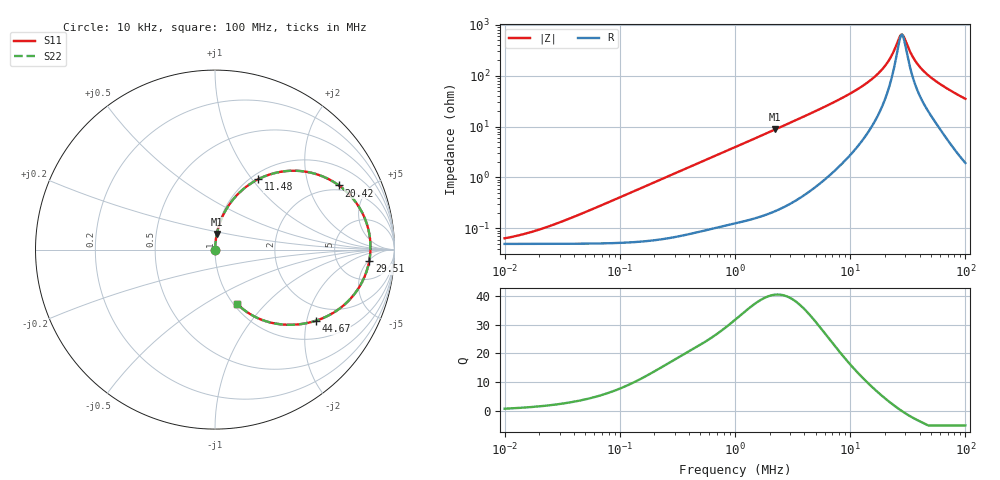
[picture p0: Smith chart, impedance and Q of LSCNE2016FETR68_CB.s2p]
! LSCNE2016FETR68_CB  S-PARAMETER MODEL  ( Standard Model )
! Model Generated by TAIYO YUDEN Corporation (http://www.ty-top.com)
! Version 1.0
! TAIYO YUDEN Control No. 200220
! Copyright(c) 2020 TAIYO YUDEN CO.,LTD. All Rights Reserved.
! Product Description (link to TY-COMPAS)
! https://ds.yuden.co.jp/TYCOMPAS/or/detail?pn=LSCNE2016FETR68MCB&u=M
! Products Name : Inductors
! Characteristics :
!  Inductance : 0.68 [uH] , SRF(min) : - [Hz] , DC Resistance(max) : 60 [mOhm]
!  Rated Current : Saturation  3.0 [A] (dL = 30 [%]), Temp Rise  2.5 [A] (dT = 40 [degC])
!  Case Size : 2.0 x 1.6 / 0.079 x 0.063 [mm/inch] , Thickness : 0.65 / 0.026 [mm/inch]
!  (Conditions: Temperature = 25 [degC] , DC Bias Current = 0 [A])
! External Node Assignments :
!  1  o---GGG---o  2
! GND o---------o GND
! Frequency Range : 10kHz  -  100MHz  [ 402 STEP ]
# MHz S RI R 50
! Freq[MHz].  S11 Real  S11 Imag  S21 Real  S21 Imag  S12 Real  S12 Imag  S22 Real  S22 Imag
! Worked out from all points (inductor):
!   401 points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, 10 kHz to 100 MHz, reference 50 ohm
!   read as one part in series: L = 641 nH near 37.15 kHz
!   highest Q = 40.4 at 2.239 MHz (marker M1), where L = 626 nH
!   self-resonance near 28.11 MHz
!   S11 on the Smith chart (normalised r, x): 10 kHz: 1.00, +0.00; 11.48 MHz: 1.08, +1.07; 20.42 MHz: 1.77, +3.20; 29.51 MHz: 11, -5; 44.67 MHz: 1.51, -2.26; 100 MHz: 1.04, -0.70
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0.01  0.000493 0.000402  0.9995 -0.000402  0.9995 -0.000402  0.000493 0.000402
0.019953  0.000494 0.000803  0.9995 -0.000803  0.9995 -0.000803  0.000494 0.000803
0.046774  0.000502 0.00188  0.9995 -0.00188  0.9995 -0.00188  0.000502 0.00188
0.218776  0.000674 0.00876  0.9993 -0.00876  0.9993 -0.00876  0.000674 0.00876
1  0.00278 0.0392  0.9972 -0.0392  0.9972 -0.0392  0.00278 0.0392
2.238721  0.00981 0.0869  0.9902 -0.0869  0.9902 -0.0869  0.00981 0.0869
4.677351  0.0392 0.1792  0.9608 -0.1792  0.9608 -0.1792  0.0392 0.1792
7.762471  0.1077 0.2876  0.8923 -0.2876  0.8923 -0.2876  0.1077 0.2876
11.48154  0.2395 0.3915  0.7605 -0.3915  0.7605 -0.3915  0.2395 0.3915
16.2181  0.4737 0.4379  0.5263 -0.4379  0.5263 -0.4379  0.4737 0.4379
20.41738  0.6908 0.3573  0.3092 -0.3573  0.3092 -0.3573  0.6908 0.3573
21.87762  0.7526 0.3024  0.2474 -0.3024  0.2474 -0.3024  0.7526 0.3024
23.98833  0.8199 0.2062  0.1801 -0.2062  0.1801 -0.2062  0.8199 0.2062
26.91535  0.864 0.0588  0.136 -0.0588  0.136 -0.0588  0.864 0.0588
28.18383  0.8661 -0.0036  0.1339 0.0036  0.1339 0.0036  0.8661 -0.0036
29.51209  0.8592 -0.0652  0.1408 0.0652  0.1408 0.0652  0.8592 -0.0652
35.48134  0.7569 -0.2714  0.2431 0.2714  0.2431 0.2714  0.7569 -0.2714
39.81072  0.6598 -0.3517  0.3402 0.3517  0.3402 0.3517  0.6598 -0.3517
44.66836  0.5601 -0.3969  0.4399 0.3969  0.4399 0.3969  0.5601 -0.3969
53.70318  0.4164 -0.4191  0.5836 0.4191  0.5836 0.4191  0.4164 -0.4191
67.6083  0.2728 -0.3957  0.7272 0.3957  0.7272 0.3957  0.2728 -0.3957
100  0.1226 -0.3017  0.8774 0.3017  0.8774 0.3017  0.1226 -0.3017
